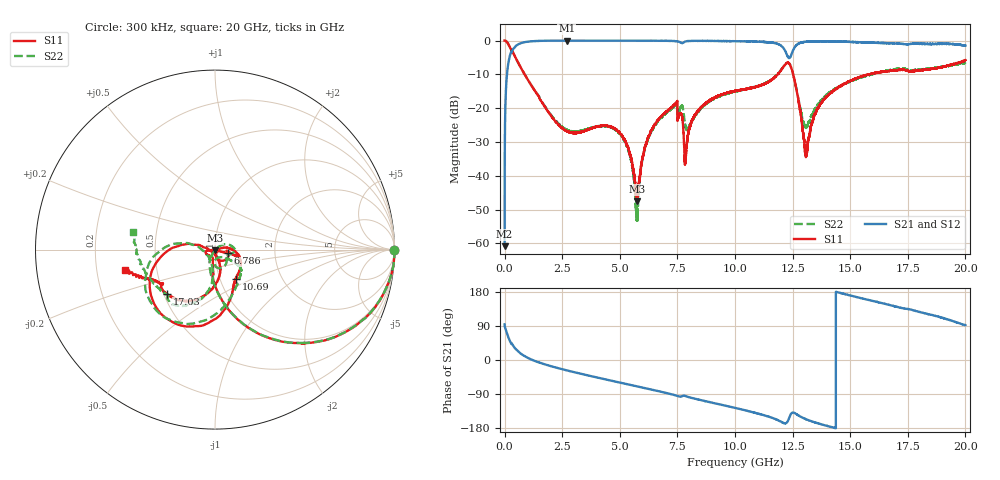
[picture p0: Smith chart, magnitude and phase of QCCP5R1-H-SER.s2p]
!QCCP5R1
!Johanson Technology Inc.
!www.johansontechnology.com
!Test Board Conditions:
!Substrate Type  RO4350B
!Substrate Thickness  20 mil
!Substrate Dk  3.66
!TL Type: GCPW
!TL Trace Width  36 mil
!TL Gap  12 mil
!Electrode orientation  Horizontal
!DUT TOPOLOGY	SERIES
!Mounting Pad LxW  26x36 mil
# MHz S  dB  R 50
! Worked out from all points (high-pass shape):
!   20001 points, 300 kHz to 20 GHz, reference 50 ohm
!   highest |S21| = -0.02 dB at 2.699 GHz (marker M1); lowest = -60.8 dB at 300 kHz (marker M2)
!   |S21| within 3 dB of the highest: 334.1 MHz to 12.18 GHz (11.84 GHz wide, 189 % of centre); 12.51 GHz to end of sweep
!   lowest |S11| = -47.5 dB at 5.749 GHz (marker M3), VSWR 1.01, Z = 49.9 - j0.414 ohm
!   |S11| at or under -10 dB: 868.7 MHz to 11.85 GHz (10.98 GHz wide, 173 % of centre); 12.52 GHz to 15.8 GHz (3.279 GHz wide, 23.2 % of centre); 15.80566 GHz to 15.81082 GHz (5.162 MHz wide, 0.0327 % of centre)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
!   |S22| runs from -53.9 to 0.0 dB; largest |S21 - S12| = 0.044
!   S11 on the Smith chart (normalised r, x): 300 kHz: open; 6.786 GHz: 1.15, -0.05; 10.69 GHz: 1.19, -0.40; 17.03 GHz: 0.52, -0.30; 20 GHz: 0.33, -0.10
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0.3  -0.00 -0.1  -60.82 93.9  -61.16 91.7  -0.00 0.0
111.298  -0.53 -21.0  -9.37 68.7  -9.38 68.8  -0.53 -21.1
303.295  -2.67 -45.1  -3.47 44.2  -3.46 44.3  -2.70 -45.1
982.285  -11.31 -83.2  -0.37 6.4  -0.36 6.3  -11.28 -83.4
2699.26  -26.78 -108.0  -0.02 -27.4  -0.03 -27.4  -26.43 -124.5
3334.25  -27.06 -129.7  -0.03 -36.7  -0.04 -36.7  -26.73 -121.6
5044.224  -27.77 -173.6  -0.04 -60.2  -0.03 -60.1  -28.01 -117.7
5749.214  -47.55 -98.5  -0.05 -69.5  -0.04 -69.7  -52.91 -24.6
6077.209  -31.78 -21.1  -0.05 -74.0  -0.06 -74.0  -32.24 38.6
6667.2  -23.49 -16.3  -0.07 -82.1  -0.08 -82.2  -23.76 28.4
6786.198  -22.57 -15.7  -0.07 -83.9  -0.09 -83.9  -22.86 25.2
7399.189  -18.77 -16.1  -0.19 -93.0  -0.18 -93.1  -19.21 2.7
7870.182  -33.54 2.7  -0.25 -95.6  -0.23 -95.6  -25.85 -81.0
8436.173  -20.57 1.3  -0.09 -104.7  -0.09 -104.7  -20.80 -35.4
10000.15  -14.90 -40.3  -0.18 -126.4  -0.21 -126.3  -15.13 -36.1
10687.14  -13.96 -54.1  -0.23 -136.5  -0.27 -136.3  -13.97 -44.3
12320.11  -6.59 -129.5  -5.11 -157.6  -5.16 -157.5  -6.65 -138.0
13053.1  -33.08 -144.2  -0.37 -155.5  -0.38 -155.4  -25.40 -146.8
13334.1  -24.57 -72.4  -0.25 -162.0  -0.26 -162.0  -22.11 -104.7
16667.05  -9.05 -130.9  -0.79 145.8  -0.70 145.0  -8.78 -120.2
17033.04  -8.75 -137.3  -0.86 140.2  -0.85 139.6  -8.38 -125.5
20000  -5.79 -167.0  -1.51 91.8  -1.32 93.6  -6.56 167.9
